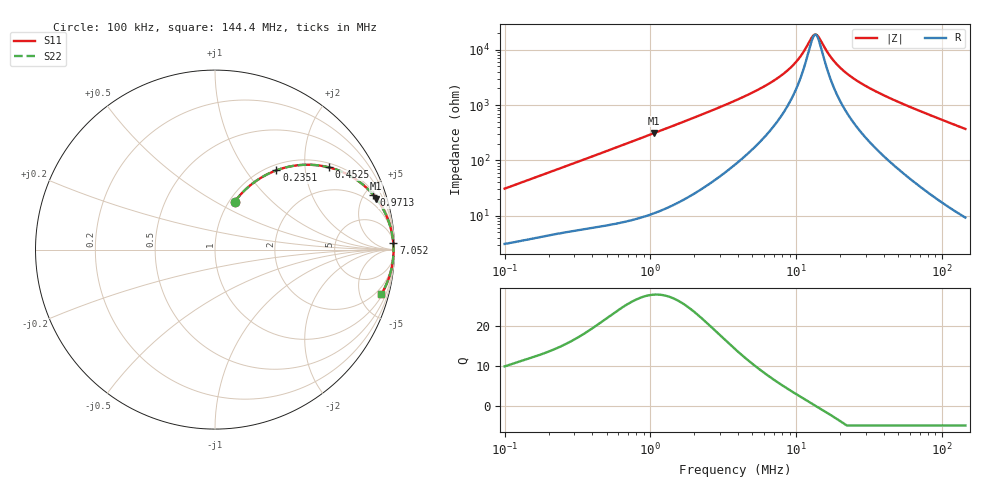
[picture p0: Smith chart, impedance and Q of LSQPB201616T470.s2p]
! LSQPB201616T470  S-PARAMETER MODEL  ( General Type )
! Model Generated by TAIYO YUDEN Corporation (http://www.ty-top.com)
! Version 2.0
! TAIYO YUDEN Control No. 100810NC14SB-FKC
! Copyright(c) 2008 TAIYO YUDEN CO.,LTD. All Rights Reserved.
! Product Description (link to TY-COMPAS)
! https://ds.yuden.co.jp/TYCOMPAS/or/detail?pn=LSQPB201616T470K&u=M
! Products Name : Inductors
! Characteristics :
!  Inductance : 47 uH , SRF(min) : 11 MHz , DC Resistance(max) : 2.86 Ohm
!  Rated Current : Saturation :210 mA , Temp Rise : 210 mA (40 degC)
!  Case Size : 2.0 x 1.6 / 0.079 x 0.063 [mm/inch] , Thickness : 1.6 / 0.063 [mm/inch]
!  (Conditions: Temperature = 25 degC , DC Bias Current/Voltage = 0A / 0V)
! External Node Assignments :
!  1  o---GGG---o  2
! GND o---------o GND
! Frequency Range : 0.1MHz  -  144.390904MHz  [ 402 STEP ]
# MHz S RI R 50
! Freq[MHz].  S11 Real  S11 Imag  S21 Real  S21 Imag  S12 Real  S12 Imag  S22 Real  S22 Imag
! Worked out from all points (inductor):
!   401 points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, 100 kHz to 144.4 MHz, reference 50 ohm
!   read as one part in series: L = 48.6 uH near 103.7 kHz
!   highest Q = 28 at 1.064 MHz (marker M1), where L = 46.8 uH
!   self-resonance near 13.33 MHz
!   S11 on the Smith chart (normalised r, x): 100 kHz: 1.06, +0.61; 235.1 kHz: 1.10, +1.41; 452.5 kHz: 1.13, +2.67; 971.3 kHz: 1.20, +5.71; 7.052 MHz: 9, +55; 144.4 MHz: 1.19, -7.41
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0.1  0.1092 0.2655  0.8908 -0.2655  0.8908 -0.2655  0.1092 0.2655
0.154729  0.2007 0.3616  0.7993 -0.3616  0.7993 -0.3616  0.2007 0.3616
0.235096  0.3425 0.4418  0.6575 -0.4418  0.6575 -0.4418  0.3425 0.4418
0.338238  0.5021 0.4727  0.4979 -0.4727  0.4979 -0.4727  0.5021 0.4727
0.452485  0.6347 0.4582  0.3653 -0.4582  0.3653 -0.4582  0.6347 0.4582
0.662949  0.7825 0.3931  0.2175 -0.3931  0.2175 -0.3931  0.7825 0.3931
0.971306  0.8822 0.3049  0.1178 -0.3049  0.1178 -0.3049  0.8822 0.3049
1.063777  0.8991 0.2839  0.1009 -0.2839  0.1009 -0.2839  0.8991 0.2839
1.144052  0.911 0.2675  0.089 -0.2675  0.089 -0.2675  0.911 0.2675
3.869624  0.9878 0.0799  0.0122 -0.0799  0.0122 -0.0799  0.9878 0.0799
7.0523  0.9934 0.035  0.00664 -0.035  0.00664 -0.035  0.9934 0.035
8.614263  0.9941 0.0234  0.0059 -0.0234  0.0059 -0.0234  0.9941 0.0234
9.963432  0.9944 0.0155  0.00556 -0.0155  0.00556 -0.0155  0.9944 0.0155
11.11225  0.9946 0.0099  0.0054 -0.0099  0.0054 -0.0099  0.9946 0.0099
12.85266  0.9947 0.00252  0.00528 -0.00252  0.00528 -0.00252  0.9947 0.00252
13.57342  0.9947 -0.000222  0.00526 0.000222  0.00526 0.000222  0.9947 -0.000222
14.07625  0.9947 -0.00205  0.00526 0.00205  0.00526 0.00205  0.9947 -0.00205
17.83085  0.9946 -0.0141  0.00543 0.0141  0.00543 0.0141  0.9946 -0.0141
22.58693  0.9941 -0.027  0.00595 0.027  0.00595 0.027  0.9941 -0.027
29.67153  0.9929 -0.0437  0.00714 0.0437  0.00714 0.0437  0.9929 -0.0437
43.47261  0.9894 -0.0728  0.0106 0.0728  0.0106 0.0728  0.9894 -0.0728
144.3909  0.9268 -0.2483  0.0732 0.2483  0.0732 0.2483  0.9268 -0.2483
